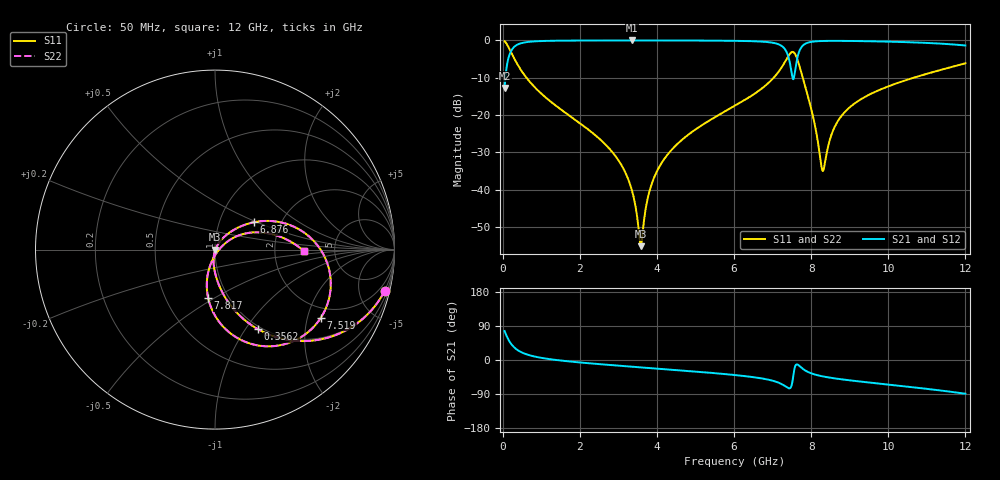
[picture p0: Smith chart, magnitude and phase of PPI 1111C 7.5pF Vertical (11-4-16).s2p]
# GHz S MA R 50
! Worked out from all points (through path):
!   1601 points, 50 MHz to 12 GHz, reference 50 ohm
!   highest |S21| = -0.02 dB at 3.359 GHz (marker M1); lowest = -12.7 dB at 50 MHz (marker M2)
!   group delay of S21, straight-line fit = 22.8 ps
!   lowest |S11| = -55.1 dB at 3.583 GHz (marker M3), VSWR 1.00, Z = 50.2 - j0.0571 ohm
!   |S11| at or under -10 dB: 616.5 MHz to 7.028 GHz (6.411 GHz wide, 168 % of centre); 7.783 GHz to 10.66 GHz (2.876 GHz wide, 31.2 % of centre)
!   |S22| runs from -55.1 to -0.2 dB; largest |S21 - S12| = 0
!   S11 on the Smith chart (normalised r, x): 50 MHz: 0.96, -8.25; 356.2 MHz: 0.96, -1.15; 6.876 GHz: 1.46, +0.48; 7.519 GHz: 1.63, -2.43; 7.817 GHz: 0.80, -0.47; 12 GHz: 2.95, -0.05
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0.05  0.9729 -13.6  0.2312 76.4  0.2312 76.4  0.9729 -13.6
0.1769688  0.7645 -41.1  0.6443 48.9  0.6443 48.9  0.7645 -41.1
0.3562187  0.5055 -61.5  0.8623 28.4  0.8623 28.4  0.5055 -61.5
0.8192812  0.2392 -80.5  0.9701 9.3  0.9701 9.3  0.2392 -80.5
2.044156  0.07489 -95.9  0.9958 -6.9  0.9958 -6.9  0.07489 -95.9
2.918  0.02849 -101.2  0.9979 -14.3  0.9979 -14.3  0.02849 -101.2
3.358656  0.009507 -97.6  0.9981 -17.7  0.9981 -17.7  0.009507 -97.6
3.582719  0.001751 -19.0  0.998 -19.4  0.998 -19.4  0.001751 -19.0
3.791844  0.008925 57.1  0.9979 -21.1  0.9979 -21.1  0.008925 57.1
4.038312  0.01923 61.3  0.9976 -22.9  0.9976 -22.9  0.01923 61.3
6.025  0.1334 48.5  0.9865 -39.7  0.9865 -39.7  0.1334 48.5
6.876437  0.2645 35.2  0.9492 -51.6  0.9492 -51.6  0.2645 35.2
7.302156  0.4949 12.0  0.7834 -67.5  0.7834 -67.5  0.4949 12.0
7.51875  0.7014 -32.7  0.3137 -54.5  0.3137 -54.5  0.7014 -32.7
7.630781  0.5787 -66.8  0.5494 -11.6  0.5494 -11.6  0.5787 -66.8
7.8175  0.2729 -98.0  0.8819 -25.8  0.8819 -25.8  0.2729 -98.0
8.019156  0.1105 -107.2  0.9588 -35.8  0.9588 -35.8  0.1105 -107.2
8.310438  0.01792 -29.3  0.9822 -43.4  0.9822 -43.4  0.01792 -29.3
8.541969  0.05737 30.0  0.9855 -47.5  0.9855 -47.5  0.05737 30.0
8.810844  0.1009 33.2  0.9848 -51.3  0.9848 -51.3  0.1009 33.2
10.01331  0.2437 23.3  0.9622 -65.0  0.9622 -65.0  0.2437 23.3
12  0.4934 -0.8  0.854 -89.0  0.854 -89.0  0.4934 -0.8
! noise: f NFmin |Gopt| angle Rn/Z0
0.05  0.0003984  0.8831  2.29  0.0007385
1.372  0.003727  0.6725  8.146  0.00218
2.701  0.006182  0.6258  14.98  0.003043
4.031  0.008625  0.6103  21.68  0.003967
5.36  0.01195  0.6302  28.18  0.005726
6.682  0.02406  0.7598  34.85  0.01851
8.012  0.0502  0.8587  41.85  0.06641
9.341  0.02447  0.702  47.31  0.01358
10.67  0.02654  0.6996  52.56  0.01401
12  0.04016  0.7767  58.34  0.02819
